PROGRAM MAIN
VAR
	// Outputs
		
	TOGGLE_RUN_ENABLE : BOOL;
	SETPOINT_PERCENT : UINT;
	
	// Inputs

	AC_LINE_VOLTAGE : UINT;
END_VAR

IF TOGGLE_RUN_ENABLE THEN
	GVL.ATOM_RUN_ENABLE := 1;
ELSE
	GVL.ATOM_RUN_ENABLE := 0;
END_IF

GVL.ATOM_SETPOINT := SETPOINT_PERCENT * 100;

AC_LINE_VOLTAGE := GVL.ATOM_AC_LINE;

END_PROGRAM
